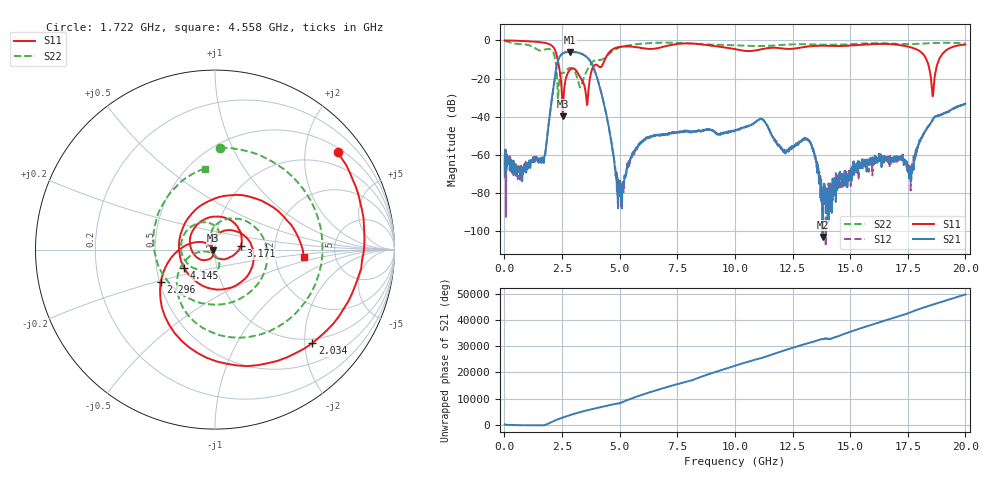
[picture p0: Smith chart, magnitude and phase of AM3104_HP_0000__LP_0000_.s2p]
!Created with skrf (http://scikit-rf.org).
# Hz S RI R 50.0
!freq ReS11 ImS11 ReS21 ImS21 ReS12 ImS12 ReS22 ImS22
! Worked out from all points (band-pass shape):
!   1601 points, 10 MHz to 20 GHz, reference 50 ohm
!   highest |S21| = -5.95 dB at 2.846 GHz (marker M1); lowest = -102.9 dB at 13.8 GHz (marker M2)
!   |S21| within 3 dB of the highest: 2.381 GHz to 3.595 GHz (1.214 GHz wide, 40.6 % of centre)
!   lowest |S11| = -39.7 dB at 2.534 GHz (marker M3), VSWR 1.02, Z = 49 - j0.31 ohm
!   |S11| at or under -10 dB: 2.313 GHz to 4.36 GHz (2.048 GHz wide, 61.4 % of centre); 18.31 GHz to 18.86 GHz (549.7 MHz wide, 2.96 % of centre)
!   |S22| runs from -31.1 to -0.2 dB; largest |S21 - S12| = 0.0048
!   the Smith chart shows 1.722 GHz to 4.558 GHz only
!   S11 on the Smith chart (normalised r, x): 1.722 GHz: 0.61, +2.75; 2.034 GHz: 0.90, -2.17; 2.296 GHz: 0.51, -0.21; 3.171 GHz: 1.33, +0.05; 4.145 GHz: 0.69, -0.14; 4.558 GHz: 2.93, -0.31
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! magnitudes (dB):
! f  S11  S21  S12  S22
! 10 MHz  0.0  -63.5  -62.9  -0.2
! 1.722 GHz  -1.2  -61.8  -62.3  -4.9
! 2.034 GHz  -2.5  -33.0  -32.9  -5.0
! 2.296 GHz  -9.1  -12.0  -12.0  -22.4
! 2.534 GHz  -39.7  -6.8  -6.8  -17.0
! 2.846 GHz  -15.3  -6.0  -6.0  -14.4
! 3.171 GHz  -16.8  -6.3  -6.2  -20.1
! 3.346 GHz  -20.5  -7.0  -7.0  -23.5
! 3.583 GHz  -33.8  -8.8  -8.8  -15.7
! 4.145 GHz  -14.0  -24.6  -24.6  -10.2
! 4.558 GHz  -6.1  -47.3  -47.5  -6.8
! 5.008 GHz  -3.4  -80.4  -74.7  -3.7
! 5.77 GHz  -3.6  -56.1  -56.2  -1.9
! 6.682 GHz  -3.9  -49.6  -49.5  -1.2
! 10.01 GHz  -4.5  -47.0  -47.3  -2.5
! 13.34 GHz  -2.9  -55.1  -56.2  -2.1
! 13.8 GHz  -2.8  -102.9  -82.4  -2.2
! 16.68 GHz  -1.8  -62.6  -63.8  -1.5
! 17.65 GHz  -3.7  -73.2  -68.9  -1.9
! 18.59 GHz  -29.2  -41.4  -41.4  -1.4
! 19.03 GHz  -6.7  -38.4  -38.4  -1.2
! 20 GHz  -2.2  -33.1  -33.2  -1.6
